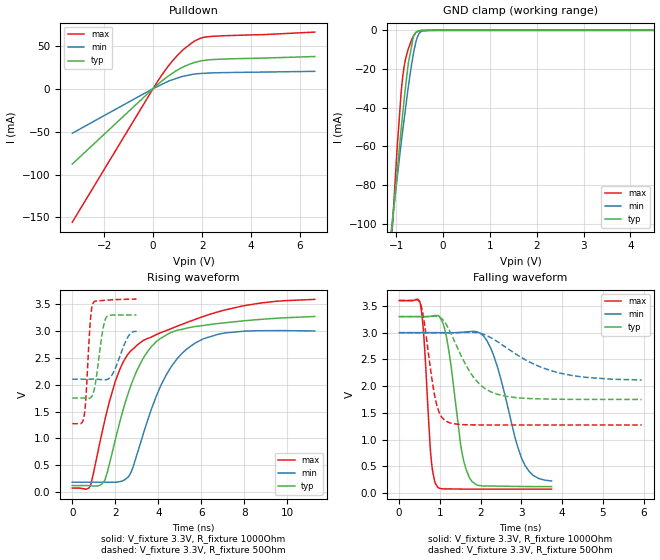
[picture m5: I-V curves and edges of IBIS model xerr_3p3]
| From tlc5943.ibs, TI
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|   xerr_3p3 Model
[Model]   xerr_3p3
Model_type   Open_drain
Polarity   Inverting
Vmeas = 1.65
Vref = 3.3
Cref = 15pF
Rref = 1000
|   typ   min   max
|   (nom PVT)   (Fast PVT)   (slow PVT)
C_comp   1.261e-12   1.253e-12   1.263e-12
|ON state : BUFFER OUTPUT TURNED LOW
|C_comp   2.474e-12   2.125e-12   2.562e-12
|OFF state: BUFFER IN HIGH IMPEDANCE
|C_comp   1.261e-12   1.253e-12   1.263e-12
| Where nom  PVT is Nominal Process,  3.3V,  65C
|   Fast PVT is Strong Process,   3.6V,  -40C
|   Slow PVT is Weak Process,   3V,  125C
[Voltage Range]   3.3   3   3.6
|Ambient Temperature   25   85   -40
|Junction Temperature
[Temperature Range]   65   125   -40
[Pullup Reference]   3.3   3   3.6
[Pulldown Reference]   0   0   0
[Power Clamp Reference]   3.3   3   3.6
[GND Clamp Reference]   0   0   0
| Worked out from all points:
|   slope of the pulldown table from 0 to 0.495 V, typ, clamps not added: 41.7 ohm
|   GND clamp passes 1 mA (typ) near -0.58 V on its own axis
|   falling waveform, V_fixture 3.3V, R_fixture 1000Ohm: 20-80 % time 325ps typ, 571ps min, 161ps max; typ from 3.3 V to 0.123 V
|   rising waveform, V_fixture 3.3V, R_fixture 1000Ohm: 20-80 % time 1.68ns typ, 1.75ns min, 2.47ns max; typ from 0.122 V to 3.27 V
|   rising waveform, V_fixture 3.3V, R_fixture 50Ohm: 20-80 % time 318ps typ, 519ps min, 198ps max; typ from 1.75 V to 3.3 V
|   falling waveform, V_fixture 3.3V, R_fixture 50Ohm: 20-80 % time 678ps typ, 1.29ns min, 267ps max; typ from 3.3 V to 1.75 V
[Pulldown]
|   Voltage   I(typ)   I(min)   I(max)
-3.3V     -87.82mA   -51.93mA   -155.5mA
172.8mV   4.455mA    2.406mA    7.955mA
478.8mV   11.52mA    6.603mA    20.79mA
741.6mV   17.04mA    9.852mA    30.52mA
1.246V    25.43mA    14.43mA    45.75mA
1.706V    30.53mA    17mA       55.61mA
1.94V     32.23mA    17.59mA    58.74mA
2.167V    33.17mA    17.95mA    60.12mA
6.6V      37.33mA    20.1mA     65.79mA
[GND Clamp]
|   Voltage   I(typ)   I(min)   I(max)
-3.3V     -806.2mA   -656.3mA   -1.136A
-1.123V   -111mA     -106.5mA   -116.9mA
-1.073V   -96.64mA   -95.14mA   -96.44mA
-986.4mV  -74.12mA   -76.94mA   -61.71mA
-896.4mV  -50.61mA   -57.95mA   -31.52mA
-838.8mV  -37.02mA   -46.92mA   -19.26mA
-745.8mV  -17.19mA   -29.26mA   -9.699mA
-633.6mV  -2.966mA   -11.79mA   -2.849mA
-544.5mV  -410.2uA   -3.098mA   -628.4uA
-462mV    -53.75uA   -406.9uA   -83.53uA
-285mV    -33.01uA   -2.598uA   -11.97uA
6.6V      0A         0A         0A
[POWER Clamp]
|   Voltage   I(typ)   I(min)   I(max)
-3.3V     0A         0A         0A
6.6V      0A         0A         0A
[Ramp]
R_load = 1000
|   typ   min   max
dV/dt_r   1.90675/1.72105e-09   1.68866/1.73878e-09   2.11487/2.50297e-09
dV/dt_f   1.90663/3.23713e-10   1.68842/5.80043e-10   2.11473/1.60611e-10
[Falling Waveform]
V_fixture = 3.3V
V_fixture_min = 3V
V_fixture_max = 3.6V
R_fixture = 1000Ohm
|   Time   V(typ)   V(min)   V(max)
0s        3.3V       3V         3.6V
520ps     3.3V       3V         3.532V
790ps     3.308V     3V         606.6mV
940ps     3.32V      3V         119.4mV
1.16ns    2.921V     2.999V     80.32mV
1.52ns    855mV      3.006V     77.01mV
1.74ns    267.7mV    3.02V      75.71mV
2.26ns    133.2mV    2.688V     75.48mV
3.09ns    125mV      518.2mV    75.52mV
3.74ns    123mV      228.3mV    75.51mV
[Rising Waveform]
V_fixture = 3.3V
V_fixture_min = 3V
V_fixture_max = 3.6V
R_fixture = 1000Ohm
|   Time   V(typ)   V(min)   V(max)
0s        122.1mV    185.4mV    75.21mV
835ps     119.4mV    185.4mV    113.3mV
1.51ns    219mV      185mV      1.334V
2.23ns    1.338V     197.1mV    2.305V
2.665ns   1.916V     318.5mV    2.606V
3.04ns    2.294V     741.7mV    2.748V
4.36ns    2.925V     2.176V     3.008V
5.725ns   3.086V     2.78V      3.219V
7.09ns    3.154V     2.965V     3.392V
11.28ns   3.272V     3.002V     3.591V
[Rising Waveform]
V_fixture = 3.3V
V_fixture_min = 3V
V_fixture_max = 3.6V
R_fixture = 50Ohm
|   Time   V(typ)   V(min)   V(max)
0s        1.752V     2.104V     1.275V
550ps     1.752V     2.104V     1.417V
640ps     1.749V     2.104V     1.798V
840ps     1.756V     2.105V     3.193V
980ps     1.852V     2.105V     3.529V
1.42ns    3.022V     2.091V     3.569V
1.57ns    3.248V     2.092V     3.574V
1.91ns    3.298V     2.227V     3.583V
2.61ns    3.3V       2.904V     3.593V
2.99ns    3.3V       2.996V     3.596V
[Falling Waveform]
V_fixture = 3.3V
V_fixture_min = 3V
V_fixture_max = 3.6V
R_fixture = 50Ohm
|   Time   V(typ)   V(min)   V(max)
0s        3.3V       3V         3.6V
520ps     3.3V       3V         3.551V
610ps     3.3V       3V         3.225V
890ps     3.307V     3V         1.754V
1.01ns    3.284V     3V         1.462V
1.16ns    3.148V     3V         1.341V
1.79ns    2.205V     3.005V     1.276V
2.31ns    1.875V     2.881V     1.275V
3.75ns    1.757V     2.284V     1.275V
5.95ns    1.752V     2.115V     1.275V
